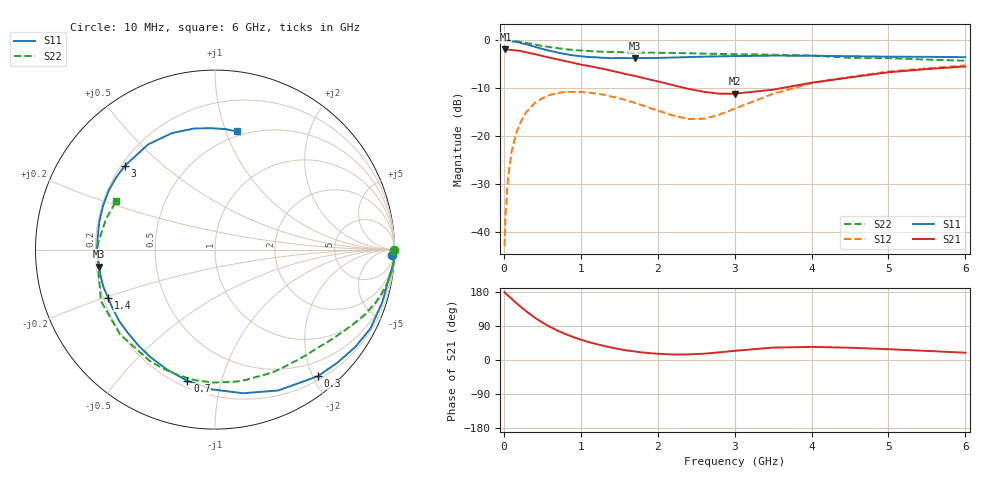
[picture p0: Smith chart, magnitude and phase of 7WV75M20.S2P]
! Infineon Technologies  Discrete & RF Semiconductors
! BFS17W
! Si NPN RF Bipolar Junction Transistor in SOT323
! VCE = 0.75 V  IC = 0.2 mA
! Common Emitter S-Parameters:  August  1999
# GHz  S  MA  R  50
!  f  S11  S21  S12  S22
! GHz  MAG  ANG  MAG  ANG  MAG  ANG  MAG  ANG
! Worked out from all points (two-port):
!   36 points, 10 MHz to 6 GHz, reference 50 ohm
!   highest |S21| = -1.84 dB at 20 MHz (marker M1); lowest = -11.1 dB at 3 GHz (marker M2)
!   |S21| within 3 dB of the highest: start of sweep to 946.6 MHz
!   lowest |S11| = -3.7 dB at 1.7 GHz (marker M3), VSWR 4.76, Z = 10.6 - j3.47 ohm
!   |S11| at or under -10 dB: nowhere
!   |S22| runs from -4.2 to 0.0 dB; largest |S21 - S12| = 0.81
!   S11 on the Smith chart (normalised r, x): 10 MHz: 26, -60; 300 MHz: 0.26, -2.07; 700 MHz: 0.24, -0.78; 1.4 GHz: 0.22, -0.21; 3 GHz: 0.21, +0.38; 6 GHz: 0.46, +1.09
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0.01  0.9879 -1.6  0.796 179.0  0.0071 87.6  0.9999 -0.2
0.02  0.9999 -3.7  0.809 176.4  0.0138 92.6  0.989 -1.3
0.05  0.9831 -8.9  0.801 170.8  0.0338 84.1  0.9974 -3.3
0.1  0.9772 -17.5  0.795 161.9  0.0685 78.5  0.9927 -6.7
0.15  0.9714 -26.9  0.787 152.5  0.1009 72.0  0.9815 -9.9
0.2  0.9514 -34.8  0.78 143.7  0.1306 67.1  0.9694 -12.8
0.3  0.9082 -51.0  0.75 127.3  0.1814 56.5  0.9409 -18.5
0.4  0.8605 -65.8  0.721 112.1  0.2215 47.0  0.9084 -23.6
0.5  0.8155 -78.9  0.689 99.2  0.2491 39.0  0.8774 -27.9
0.7  0.7469 -101.9  0.634 77.4  0.2821 26.2  0.8305 -35.6
0.9  0.6993 -120.7  0.585 60.7  0.2907 16.5  0.7951 -42.8
1.1  0.6716 -136.4  0.542 47.4  0.2858 8.9  0.7753 -49.8
1.4  0.6532 -155.6  0.482 32.8  0.2594 1.0  0.7584 -60.6
1.7  0.6525 -171.7  0.427 22.6  0.2234 -2.5  0.7456 -72.0
2.2  0.6632 166.2  0.341 14.5  0.1642 6.0  0.7405 -90.9
2.6  0.6775 150.9  0.291 16.6  0.1521 27.4  0.7289 -106.3
3  0.6863 137.2  0.278 24.2  0.1937 44.4  0.7186 -120.6
3.5  0.6942 122.4  0.306 32.7  0.277 49.1  0.7092 -138.4
4  0.6919 110.3  0.362 34.6  0.358 44.9  0.697 -155.9
4.5  0.6847 99.8  0.411 32.4  0.4166 38.8  0.6579 -171.1
5.5  0.674 85.2  0.502 24.0  0.5119 27.0  0.6308 164.4
6  0.669 79.6  0.535 19.2  0.5482 21.5  0.6136 153.8
